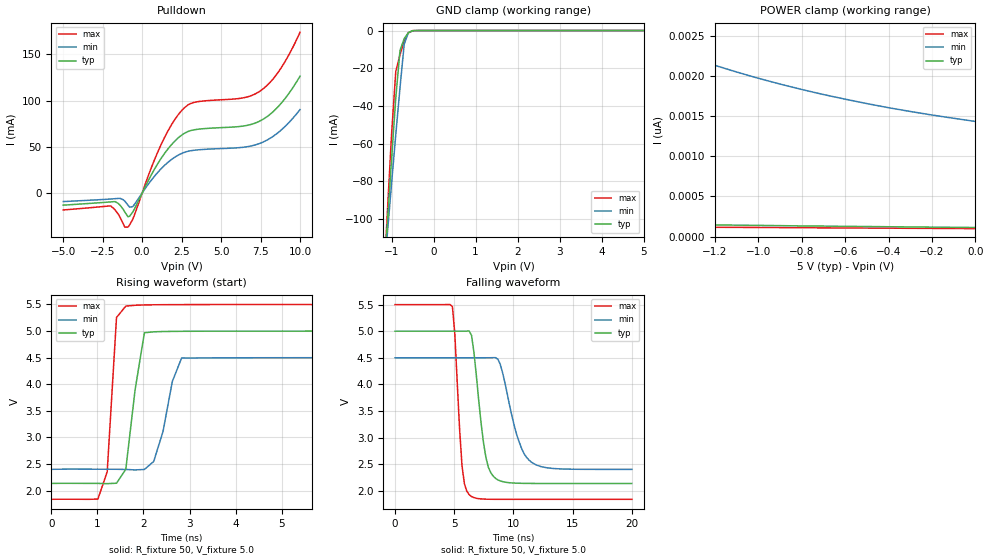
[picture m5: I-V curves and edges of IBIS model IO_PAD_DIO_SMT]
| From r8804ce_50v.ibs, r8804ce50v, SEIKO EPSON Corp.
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[Model]   IO_PAD_DIO_SMT
Model_type I/O_open_drain
Enable Active-High
Polarity Non-Inverting
Vinh=4.4
Vinl=0.9
Vref=5.5
Vmeas=2.5
Rref=5000
C_comp   2.5p   2.0p   3.0p
[Temperature Range] 25   105   -40
[Voltage Range]   5.0   4.5   5.5
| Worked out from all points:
|   slope of the pulldown table from 0 to 0.75 V, typ, clamps not added: 30.2 ohm
|   GND clamp passes 1 mA (typ) near -0.59 V on its own axis
|   falling waveform, R_fixture 50, V_fixture 5.0: 20-80 % time 868ps typ, 1.42ns min, 537ps max; typ from 5 V to 2.14 V
|   rising waveform, R_fixture 50, V_fixture 5.0: 20-80 % time 260ps typ, 319ps min, 153ps max; typ from 2.14 V to 5 V
[Pulldown]
-5V       -13.17mA   -9.281mA   -18.37mA
-2V       -9.661mA   -6.523mA   -13.97mA
-1.5V     -11.48mA   -5.863mA   -23.2mA
-1.1V     -20.65mA   -8.791mA   -36.89mA
-900mV    -25.65mA   -13.16mA   -36.97mA
-600mV    -20.79mA   -14.82mA   -28.65mA
1.1V      34.77mA    24.37mA    48.65mA
2.4V      61.28mA    41.98mA    87.21mA
3.3V      68.39mA    46.26mA    98.05mA
7.4V      77.39mA    53.31mA    109.5mA
8.6V      93.1mA     65.15mA    130.2mA
10V       126.3mA    90.21mA    173.8mA
[GND Clamp]
-5V       -1.481A    -1.201A    -1.847A
-1.2V     -136mA     -134.3mA   -139.6mA
-1.1V     -101.9mA   -107.5mA   -96.17mA
-1V       -68.06mA   -80.96mA   -54.69mA
-900mV    -35.73mA   -55.1mA    -21.63mA
-800mV    -10.6mA    -30.38mA   -12.89mA
-700mV    -4.3mA     -7.212mA   -5.615mA
-600mV    -1.094mA   -1.181mA   -1.208mA
-500mV    -109.6uA   -173.5uA   -67.33uA
-400mV    -6.015uA   -18.81uA   -1.378uA
5V        112.6pA    1.656nA    89.7pA
[POWER Clamp]
-5V       435pA      13.27nA    172.1pA
-4.4V     357.7pA    10.02nA    161.9pA
-3.5V     268.5pA    6.437nA    147.8pA
-2.7V     212.6pA    4.294nA    136.2pA
-1.7V     163.5pA    2.645nA    122.6pA
-1.6V     159.6pA    2.529nA    121.9pA
-1.4V     152.6pA    2.318nA    117.3pA
-1.2V     144.4pA    2.133nA    114.8pA
-1V       138.9pA    1.972nA    112.8pA
-800mV    132.1pA    1.833nA    110.3pA
-400mV    122pA      1.605nA    104.4pA
0V        112.6pA    1.434nA    98pA
[Falling Waveform]
R_fixture=50
V_fixture=5.0
V_fixture_min=4.5
V_fixture_max=5.5
0s        5V         4.5V       5.5V
4.848ns   5V         4.5V       5.463V
5.657ns   5V         4.5V       2.473V
6.263ns   5.004V     4.5V       1.924V
6.667ns   4.601V     4.5V       1.87V
7.677ns   2.625V     4.5V       1.84V
8.485ns   2.232V     4.502V     1.838V
10.3ns    2.141V     3.034V     1.837V
11.52ns   2.136V     2.536V     1.837V
20ns      2.136V     2.401V     1.837V
[Rising Waveform]
R_fixture=50
V_fixture=5.0
V_fixture_min=4.5
V_fixture_max=5.5
0s        2.136V     2.401V     1.837V
1.01ns    2.136V     2.403V     1.842V
1.212ns   2.131V     2.402V     2.355V
1.414ns   2.139V     2.402V     5.255V
1.616ns   2.403V     2.398V     5.47V
1.818ns   3.9V       2.39V      5.486V
2.02ns    4.969V     2.398V     5.492V
2.222ns   4.987V     2.549V     5.494V
2.828ns   4.996V     4.495V     5.498V
20ns      5V         4.5V       5.5V
[Ramp]
R_load=50
dV/dt_r   1.719E+0/1.939E-10   1.260E+0/2.916E-10   2.198E+0/1.450E-10
dV/dt_f   1.719E+0/8.533E-10   1.260E+0/1.408E-9   2.198E+0/5.259E-10
|[End   IO_PAD_DIO_SMT
